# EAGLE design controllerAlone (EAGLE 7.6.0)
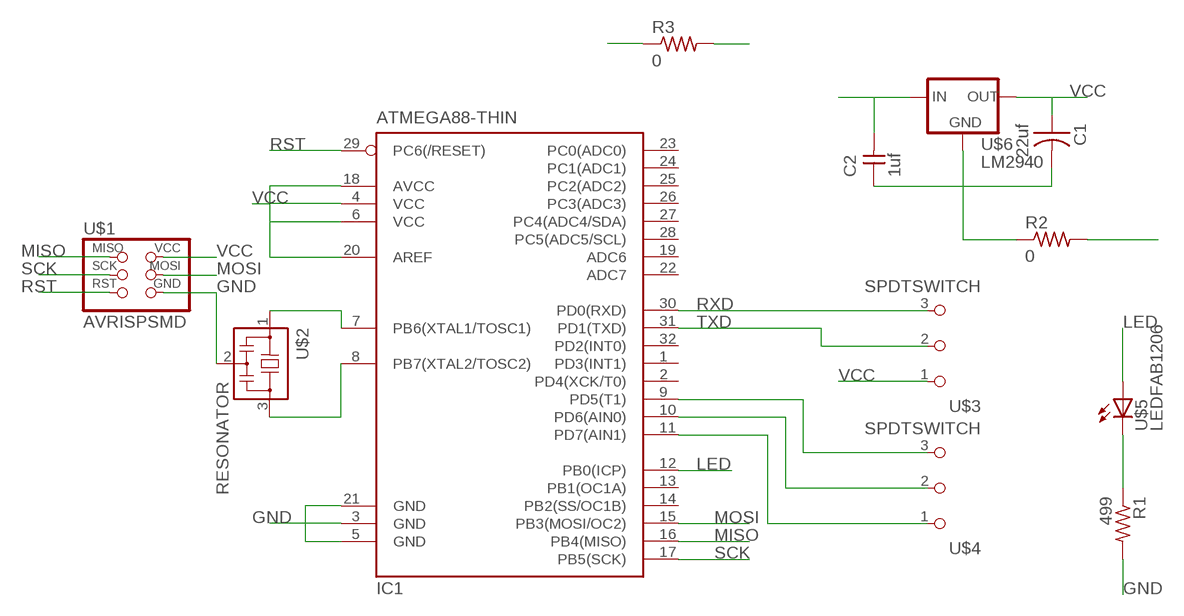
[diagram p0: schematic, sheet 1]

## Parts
C1  22uf  CAP-US1206FAB  [C1206FAB]
C2  1uf  CAP-UNPOLARIZEDFAB  [C1206FAB]
IC1  ATMEGA88-THIN  [TQFP32-08THIN]
R1  499  RES-US1206FAB  [R1206FAB]
R2  0  RES-US1206FAB  [R1206FAB]
R3  0  RES-US1206FAB  [R1206FAB]
U$1  AVRISPSMD  [2X03SMD]
U$2  RESONATOR  [EFOBM]
U$3  SPDTSWITCH  [SPDTSWITCH]
U$4  SPDTSWITCH  [SPDTSWITCH]
U$5  LEDFAB1206  [LED1206FAB]
U$6  LM2940  V_REG_MIC2920  [SOT223]

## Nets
GND: C1.2 C2.1 IC1.3(GND) IC1.5(GND) IC1.21(GND) R1.2 R2.1 R2.2 U$1.6(GND) U$2.2 U$6.2(GND)
LED: IC1.12(PB0(ICP)) U$5.1(A)
MISO: IC1.16(PB4(MISO)) U$1.1(MISO)
MOSI: IC1.15(PB3(MOSI/OC2)) U$1.4(MOSI)
N$1: IC1.9(PD5(T1)) U$4.3
N$2: IC1.10(PD6(AIN0)) U$4.2
N$3: IC1.11(PD7(AIN1)) U$4.1
N$4: C2.2 U$6.1(IN)
N$7: R1.1 U$5.2(C)
N$9: IC1.7(PB6(XTAL1/TOSC1)) U$2.1
N$10: IC1.8(PB7(XTAL2/TOSC2)) U$2.3
RST: IC1.29(PC6(/RESET)) U$1.5(RST)
RXD: IC1.30(PD0(RXD)) U$3.3
SCK: IC1.17(PB5(SCK)) U$1.3(SCK)
TXD: IC1.31(PD1(TXD)) U$3.2
VCC: C1.1 IC1.4(VCC) IC1.6(VCC) IC1.18(AVCC) IC1.20(AREF) R3.1 R3.2 U$1.2(VCC) U$3.1 U$6.3(OUT)
Unconnected: IC1.1(PD3(INT1)) IC1.2(PD4(XCK/T0)) IC1.13(PB1(OC1A)) IC1.14(PB2(SS/OC1B)) IC1.19(ADC6) IC1.22(ADC7) IC1.23(PC0(ADC0)) IC1.24(PC1(ADC1)) IC1.25(PC2(ADC2)) IC1.26(PC3(ADC3)) IC1.27(PC4(ADC4/SDA)) IC1.28(PC5(ADC5/SCL)) IC1.32(PD2(INT0))

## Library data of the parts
C1 = fab:CAP-US
C2 = fab:CAP-UNPOLARIZED
IC1 = fab:ATMEGA88-THIN
R1-R3 = fab:RES-US: Resistor (US Symbol)
U$1 = fab:AVRISP
U$2 = fab:RESONATOR
U$3 U$4 = fab:SPDTSWITCH
U$5 = fab:LED: LED
U$6 = SparkFun-PowerIC:V_REG_MIC2920: MIC2920A (http://www.micrel.com/_PDF/mic2920.pdf) - 400mA output LDO Regulator

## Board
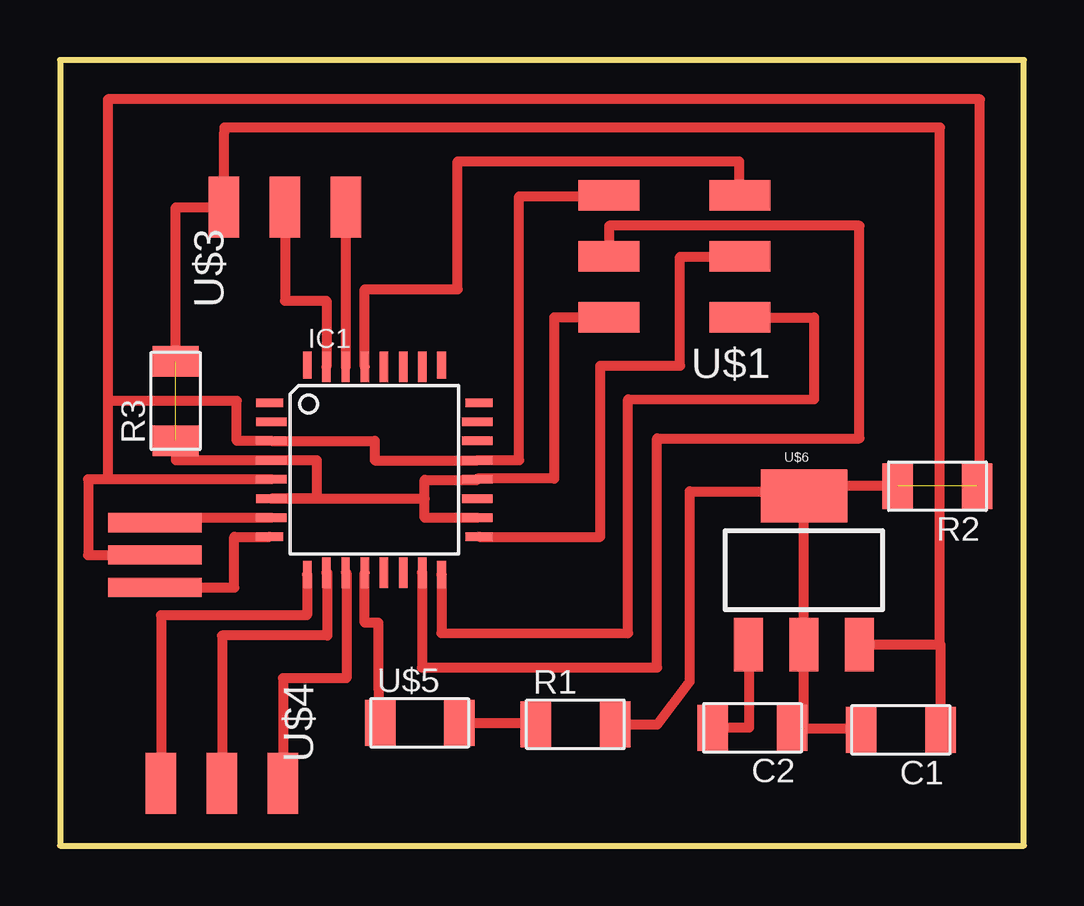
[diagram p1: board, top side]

Size 40.18 x 32.76 mm. Coordinates in mm from the lower left corner, seen from the top.
Outline: 0,0 40.18,0 40.18,32.76 0,32.76 0,0
Copper layers (1*16): Top 0.035mm / dielectric 1.5mm / Bottom 0.035mm
Design rules "default *": minimum track width 16mil, minimum drill 24mil, track to track 16mil, track to pad 16mil, pad to pad 8mil, via to via 8mil, smd to smd 8mil, copper to edge 40mil, drill to drill 8mil, minimum pad ring 10mil, minimum via ring 8mil, stop-mask expansion 4mil, vias tented up to drill 0mil, thermal gap 10mil

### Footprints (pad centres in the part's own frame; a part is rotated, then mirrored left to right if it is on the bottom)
C1206FAB = smd 1.27 x 1.905: 1 -1.651,0; 2 1.651,0
TQFP32-08THIN = smd 1.118 x 0.356: 1 -4.369,2.8; 8 -4.369,-2.8; 17 4.369,-2.8; 24 4.369,2.8 | smd 1.27 x 0.356: 2 -4.293,2; 3 -4.293,1.2; 4 -4.293,0.4; 5 -4.293,-0.4; 6 -4.293,-1.2; 7 -4.293,-2; 18 4.293,-2; 19 4.293,-1.2; 20 4.293,-0.4; 21 4.293,0.4; 22 4.293,1.2; 23 4.293,2 | smd 0.356 x 1.118: 9 -2.8,-4.369; 16 2.8,-4.369; 25 2.8,4.369; 32 -2.8,4.369 | smd 0.356 x 1.27: 10 -2,-4.293; 14 1.2,-4.293; 15 2,-4.293; 26 2,4.293; 27 1.2,4.293; 31 -2,4.293 | smd 0.35 x 1.27: 11 -1.2,-4.293; 12 -0.4,-4.293; 13 0.4,-4.293; 28 0.4,4.293; 29 -0.4,4.293; 30 -1.2,4.293
R1206FAB = smd 1.27 x 1.905: 1 -1.651,0; 2 1.651,0
2X03SMD = smd 2.54 x 1.27: 1 -2.54,2.54; 2 2.92,2.54; 3 -2.54,0; 4 2.92,0; 5 -2.54,-2.54; 6 2.92,-2.54
EFOBM = smd 0.8 x 3.9: 1 -1.35,0; 2 0,0; 3 1.35,0
SPDTSWITCH = smd 2.54 x 1.27: 1 0.38,2.54; 2 0.38,0; 3 0.38,-2.54
LED1206FAB = smd 1.27 x 1.905: 1 -1.651,0; 2 1.651,0
SOT223 = smd 1.219 x 2.235: 1 -2.311,-3.099; 2 0,-3.099; 3 2.311,-3.099 | smd 3.6 x 2.2: 4 0,3.099

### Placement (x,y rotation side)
C1  35.05,4.83 180 top
C2  28.87,4.91 180 top
IC1  13.11,15.67 0 top
R1  21.49,5.05 0 top
R2  36.58,14.99 180 top
R3  4.83,18.54 90 top
U$1  25.81,24.56 180 top
U$2  3.96,12.12 270 top
U$3  9.37,26.24 90 top
U$4  6.76,2.97 270 top
U$5  15,5.12 0 top
U$6  31.01,11.48 0 top

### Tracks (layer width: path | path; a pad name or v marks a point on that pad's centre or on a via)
GND  (2 unrouted)
  Top 0.406: IC1.5 1.99,15.27 | 1.99,15.27 1.17,15.27 1.17,12.12 U$2.2 | U$1.6 22.89,27.08 19.14,27.08 19.14,16.07 IC1.21 13.12,16.07 13.12,16.87 IC1.3 7.37,16.87 7.37,18.54 1.99,18.54 | 31,4.89 31,14.77 | R1.2 24.91,5.05 26.25,6.84 26.25,14.77 31,14.77 | R2.2 31,14.99 31,14.77 | C2.1 31.01,4.89 | 31.01,4.89 U$6.2 | 31.01,4.89 33.4,4.89 C1.2 | R2.1 38.35,14.99 38.35,31.11 1.99,31.11 1.99,18.54 | 1.99,18.54 1.99,15.27
LED
  Top 0.406: U$5.1 13.27,6.72 13.27,9.3 12.71,9.3 IC1.12
MISO
  Top 0.406: U$1.1 31.45,22.02 31.45,18.62 23.69,18.61 23.69,8.85 15.9,8.87 IC1.16
MOSI
  Top 0.406: IC1.15 15.09,11.38 15.09,7.43 24.89,7.43 24.89,16.98 33.33,16.98 33.33,25.84 22.89,25.84 U$1.4
N$1
  Top 0.406: IC1.9 10.3,9.6 4.22,9.6 U$4.3
N$2
  Top 0.406: IC1.10 11.14,11.38 11.14,8.76 6.76,8.76 U$4.2
N$3
  Top 0.406: IC1.11 11.94,11.38 11.94,6.99 9.3,6.99 U$4.1
N$4
  Top 0.406: U$6.1 28.73,8.38 28.73,4.92 C2.2
N$7
  Top 0.406: U$5.2 19.84,5.12 R1.1
N$9
  Top 0.406: IC1.7 3.96,13.67 U$2.1
N$10
  Top 0.406: U$2.3 7.26,10.77 7.26,12.88 IC1.8
RST
  Top 0.406: IC1.29 12.71,23.2 16.57,23.2 16.57,28.54 28.31,28.54 28.31,27.1 U$1.5
RXD
  Top 0.406: U$3.3 IC1.30
SCK
  Top 0.406: IC1.17 22.53,12.87 22.53,20.02 25.84,20.02 25.84,24.55 28.35,24.55 U$1.3
TXD
  Top 0.406: U$3.2 9.38,26.62 9.38,22.72 11.11,22.72 IC1.31
VCC  (1 unrouted)
  Top 0.406: 15.2,14.47 IC1.6 10.71,14.46 10.71,16.07 IC1.4 4.83,16.07 R3.1 | 15.2,14.47 15.2,15.25 17.4,15.25 IC1.20 17.4,15.3 20.6,15.3 20.6,22.02 U$1.2 | IC1.18 15.2,13.67 15.2,14.47 | U$6.3 36.68,8.38 | 36.68,8.38 36.68,29.93 6.84,29.93 6.84,29.74 6.84,27.11 6.84,26.62 U$3.1 4.83,26.62 R3.2 | 36.68,8.38 36.7,8.38 C1.1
